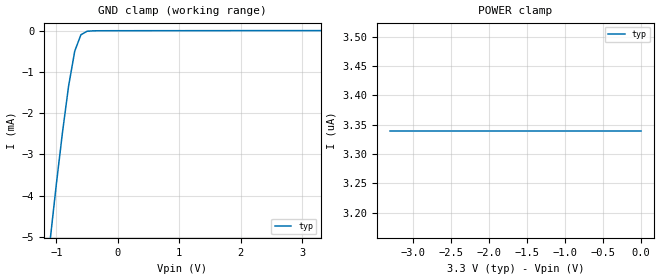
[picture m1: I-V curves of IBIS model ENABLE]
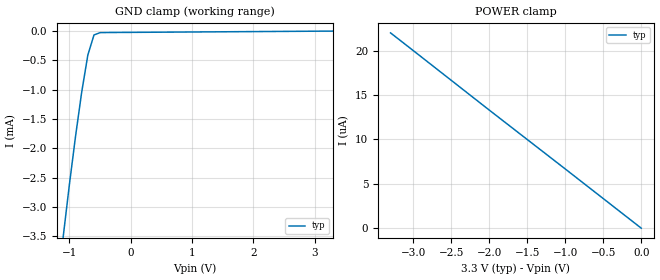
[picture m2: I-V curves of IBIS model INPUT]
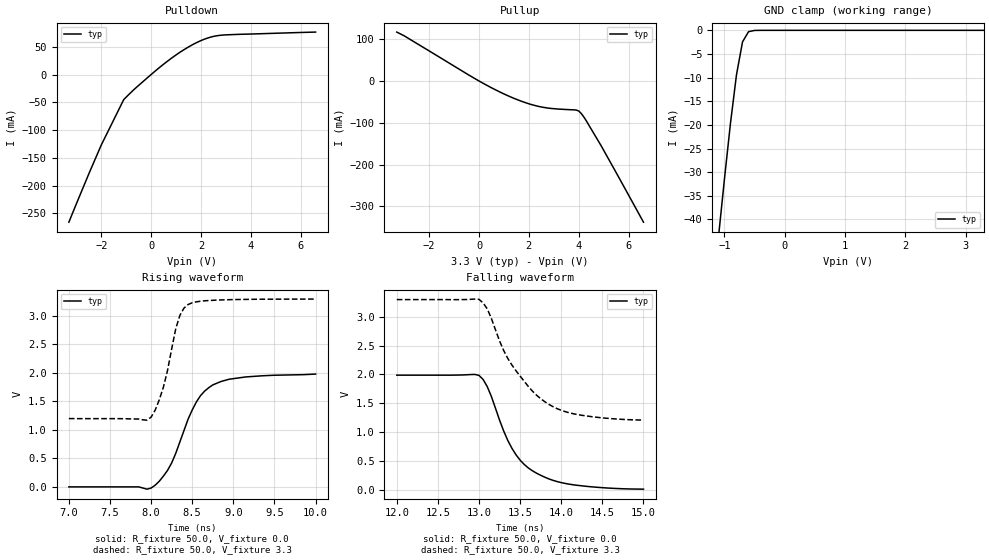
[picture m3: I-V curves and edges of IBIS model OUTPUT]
|   Texas Instruments Incorporated
|   Data Transmissions Products
|   IBIS Model for SN65LVDT386
|   64DGG TSSOP Package
[IBIS Ver]   2.1
[Comment char]   |_char
[File name]   lvdt386.ibs
[File Rev]   1.0
[Date]   28Jul99
[Source]   File originated at Texas Instruments Incorporated.
   Data Transmission Products Group.
[Notes]
[Disclaimer]
(C) Copyright Texas Instruments Incorporated 1999
   All rights reserved
  Texas Instruments Incorporated hereby grants the user of this IBIS
model a non-exclusive, nontransferable license to use this IBIS model
under the following terms.  Before using this IBIS model, the user
should read this license.  If the user does not accept these terms,
the IBIS model should be returned to Texas Instruments within 30 days.
  The user is granted this license only to use the IBIS model and
is not granted rights to sell, load, rent, lease or license the IBIS
model in whole or in part, or in modified form to anyone other than
user.  User may modify the IBIS model to suit its specific applications
but rights to derivative works and such modifications shall belong to
Texas Instruments.
  This IBIS model is provided on an "AS IS" basis and Texas Instruments
makes absolutely no warranty with respect to the information contained
herein.  TEXAS INSTRUMENTS DISCLAIMS AND CUSTOMER WAIVES ALL WARRANTIES,
EXPRESS OR IMPLIED, INCLUDING WARRANTIES OF MERCHANTABILITY OR FITNESS
FOR A PARTICULAR PURPOSE. The entire risk as to quality and performance
is with the Customer. ACCORDINGLY, IN NO EVENT SHALL THE COMPANY BE LIABLE
FOR ANY DAMAGES, WHETHER IN CONTRACT OR TORT,INCLUDING ANY LOST PROFITS
OR OTHER INCIDENTAL, CONSEQUENTIAL, EXEMPLARY, OR PUNITIVE DAMAGES ARISING
OUT OF THE USE OR APPLICATION OF THE IBIS model provided in this package.
Further, Texas Instruments reserves the right to discontinue or make changes
without notice to any product herein to improve reliability, function, or
design. Texas Instruments does not convey any license under patent rights
or any other intellectual property rights, including those of third parties.
Contact Texas Instruments at ATTN:DATA TRANSMISSIONS
Thomas Fisher 8505 Forest Lane, M/S 8710, Dallas, TX 75243-4136
[Copyright]   Copyright 1999, Texas Instruments, All Rights Reserved
[Component]   LVDT386DGG
[Manufacturer]  Texas Instruments Incorporated
[Package]
|   typ   min   max
R_pkg   0.068   0.046   0.094
L_pkg   3.798nH   2.565nH   5.991nH
C_pkg   0.564pF   0.297pF   1.022pF
[Pin]   signal_name   model_name   R_pin   L_pin   C_pin
1   A1A   INPUT   0.094   5.991n   0.940p
2   A1B   INPUT   0.090   5.514n   1.005p
3   A2A   INPUT   0.092   5.261n   0.912p
4   A2B   INPUT   0.092   4.891n   0.805p
5   A3A   INPUT   0.085   4.561n   0.702p
6   A3B   INPUT   0.084   4.247n   0.597p
7   A4A   INPUT   0.080   3.933n   0.534p
8   A4B   INPUT   0.077   3.622n   0.523p
9   B1A   INPUT   0.050   3.372n   0.483p
10   B1B   INPUT   0.048   3.139n   0.415p
11   B2A   INPUT   0.049   3.042n   0.397p
12   B2B   INPUT   0.051   2.941n   0.384p
13   B3A   INPUT   0.050   2.800n   0.355p
14   B3B   INPUT   0.052   2.711n   0.335p
15   B4A   INPUT   0.051   2.589n   0.314p
16   B4B   INPUT   0.055   2.604n   0.303p
17   C1A   INPUT   0.055   2.597n   0.302p
18   C1B   INPUT   0.052   2.605n   0.315p
19   C2A   INPUT   0.051   2.694n   0.334p
20   C2B   INPUT   0.050   2.772n   0.352p
21   C3A   INPUT   0.048   2.864n   0.372p
22   C3B   INPUT   0.049   2.982n   0.392p
23   C4A   INPUT   0.049   3.129n   0.413p
24   C4B   INPUT   0.046   3.263n   0.480p
25   D1A   INPUT   0.077   3.592n   0.542p
26   D1B   INPUT   0.081   3.923n   0.557p
27   D2A   INPUT   0.086   4.252n   0.614p
28   D2B   INPUT   0.085   4.525n   0.714p
29   D3A   INPUT   0.087   4.810n   0.813p
30   D3B   INPUT   0.089   5.135n   0.918p
31   D4A   INPUT   0.090   5.486n   1.019p
32   D4B   INPUT   0.090   5.912n   0.936p
33   GND   GND   0.087   5.926n   0.931p
34   VCC   POWER   0.087   5.496n   1.004p
35   VCC   POWER   0.087   5.124n   0.902p
36   GND   GND   0.088   4.867n   0.807p
37   END   ENABLE   0.086   4.514n   0.707p
38   D4Y   OUTPUT   0.085   4.206n   0.605p
39   D3Y   OUTPUT   0.089   3.929n   0.537p
40   D2Y   OUTPUT   0.079   3.584n   0.528p
41   D1Y   OUTPUT   0.048   3.299n   0.481p
42   ENC   ENABLE   0.048   3.101n   0.409p
43   C4Y   OUTPUT   0.048   2.969n   0.388p
44   C3Y   OUTPUT   0.048   2.855n   0.369p
45   C2Y   OUTPUT   0.049   2.766n   0.349p
46   C1Y   OUTPUT   0.051   2.696n   0.331p
47   GND   GND   0.052   2.638n   0.315p
48   VCC   POWER   0.053   2.565n   0.297p
49   VCC   POWER   0.052   2.574n   0.299p
50   GND   GND   0.051   2.617n   0.313p
51   B4Y   OUTPUT   0.050   2.666n   0.329p
52   B3Y   OUTPUT   0.050   2.769n   0.350p
53   B2Y   OUTPUT   0.049   2.909n   0.378p
54   B1Y   OUTPUT   0.048   2.993n   0.390p
55   ENB   ENABLE   0.049   3.176n   0.416p
56   A4Y   OUTPUT   0.048   3.295n   0.483p
57   A3Y   OUTPUT   0.079   3.569n   0.536p
58   A2Y   OUTPUT   0.082   3.908n   0.547p
59   A1Y   OUTPUT   0.086   4.238n   0.613p
60   ENA   ENABLE   0.086   4.509n   0.714p
61   GND   GND   0.089   4.863n   0.822p
62   VCC   POWER   0.090   5.197n   0.923p
63   VCC   POWER   0.092   5.558n   1.022p
64   GND   GND   0.090   5.947n   0.946p
[Diff_pin]   inv_pin   vdiff   tdelay_typ   tdelay_min   tdelay_max
| The 'xA' pin is Diff_pin and the 'xB' pin is the inv_pin
1   2   100   0 0 0
3   4   100   0 0 0
5   6   100   0 0 0
7   8   100   0 0 0
9   10   100   0 0 0
11   12   100   0 0 0
13   14   100   0 0 0
15   16   100   0 0 0
17   18   100   0 0 0
19   20   100   0 0 0
21   22   100   0 0 0
23   24   100   0 0 0
25   26   100   0 0 0
27   28   100   0 0 0
29   30   100   0 0 0
31   32   100   0 0 0
| Models and submodels in the file (3): ENABLE (Input), INPUT (Input), OUTPUT (3-state)
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|   Enable Model
[Model]   ENABLE
Model_type   Input
|Signals   ENA,ENB,ENC,END
Vinh = 2.0
Vinl = 0.8
|   typ   min   max
C_comp   1.0pF   NA   NA
|   typ   min   max
[Temperature Range]   25.0   NA   NA
[Voltage range]   3.3V   3.0V   3.6V
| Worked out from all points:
|   GND clamp passes 1 mA (typ) near -0.76 V on its own axis
[GND_clamp]
|   Voltage   I(typ)   I(min)   I(max)
-3.3V     -43.1mA    NA         NA
-1.1V     -5.08mA    NA         NA
-1V       -3.73mA    NA         NA
-900mV    -2.47mA    NA         NA
-800mV    -1.34mA    NA         NA
-700mV    -493uA     NA         NA
-600mV    -98.5uA    NA         NA
-500mV    -13.3uA    NA         NA
3.3V      3.34uA     NA         NA
[Power_clamp]
| Note that the[POWER_clamp]voltage table is referenced to Vcc
| and is calculated using Vtable=Vcc - Vmeasured.
|   Voltage   I(typ)   I(min)   I(max)
-3.3V     3.34uA     NA         NA
-2.7V     3.34uA     NA         NA
-2V       3.34uA     NA         NA
-800mV    3.34uA     NA         NA
0V        3.34uA     NA         NA
|   Receiver Input Model
[Model]   INPUT
Model_type   Input
|Signals   A1A,A1B,A2A,A2B,A3A,A3B,A4A,A4B,B1A,B1B,B2A,B2B,B3A,B3B,B4A,B4B
|   C1A,C1B,C2A,C2B,C3A,C3B,C4A,C4B,D1A,D1B,D2A,D2B,D3A,D3B,D4A,D4B
Vinh = 2.0
Vinl = 0.8
|   typ   min   max
C_comp   1.0pF   NA   NA
|   typ   min   max
[Temperature Range]   25.0   NA   NA
[Voltage range]   3.3V   3.0V   3.6V
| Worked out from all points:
|   GND clamp passes 1 mA (typ) near -0.79 V on its own axis
[GND_clamp]
|   Voltage   I(typ)   I(min)   I(max)
-3.3V     -32.7mA    NA         NA
-1.1V     -3.49mA    NA         NA
-1V       -2.61mA    NA         NA
-900mV    -1.79mA    NA         NA
-800mV    -1.04mA    NA         NA
-700mV    -409uA     NA         NA
-600mV    -66.6uA    NA         NA
-500mV    -26.4uA    NA         NA
3.3V      40.7pA     NA         NA
[Power_clamp]
| Note that the[POWER_clamp]voltage table is referenced to Vcc
| and is calculated using Vtable=Vcc - Vmeasured.
|   Voltage   I(typ)   I(min)   I(max)
-3.3V     22uA       NA         NA
-3V       20uA       NA         NA
-2V       13.3uA     NA         NA
-1V       6.67uA     NA         NA
0V        40.7pA     NA         NA
|   Receiver Output Model
[Model]   OUTPUT
Model_type   3-state
| Signals   A1Y,A2Y,B1Y,B2Y,C1Y,C2Y,D1Y,D2Y
Vmeas = 1.5V   |Reference voltage for timing measurements
Cref = 8pF   |Timing specification test load capacitance value
Vref = 0   |Timing specification test load voltage; GND
| variable   typ   min   max
C_comp   1.0pF   NA   NA
|   typ   min   max
[Temperature Range]   25.0   NA   NA
[Voltage range]   3.3V   3.0V   3.6V
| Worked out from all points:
|   slope of the pulldown table from 0 to 0.495 V, typ, clamps not added: 26.9 ohm
|   slope of the pullup table from 0 to 0.495 V, typ, clamps not added: 30.7 ohm
|   GND clamp passes 1 mA (typ) near -0.63 V on its own axis
|   rising waveform, R_fixture 50.0, V_fixture 0.0: 20-80 % time 352ps typ, NA min, NA max; typ from 0 V to 1.98 V
|   falling waveform, R_fixture 50.0, V_fixture 0.0: 20-80 % time 420ps typ, NA min, NA max; typ from 1.99 V to 0.006 V
|   rising waveform, R_fixture 50.0, V_fixture 3.3: 20-80 % time 202ps typ, NA min, NA max; typ from 1.2 V to 3.3 V
|   falling waveform, R_fixture 50.0, V_fixture 3.3: 20-80 % time 538ps typ, NA min, NA max; typ from 3.3 V to 1.21 V
[Pulldown]
|   Voltage   I(typ)   I(min)   I(max)
-3.3V     -266mA     NA         NA
-2.5V     -179mA     NA         NA
-2V       -127mA     NA         NA
-1.1V     -45.3mA    NA         NA
-600mV    -23.5mA    NA         NA
600mV     22.1mA     NA         NA
1.2V      41.4mA     NA         NA
1.7V      54.7mA     NA         NA
2.1V      63mA       NA         NA
2.5V      68.7mA     NA         NA
3V        71.5mA     NA         NA
6.6V      76.5mA     NA         NA
[Pullup]
|   Voltage   I(typ)   I(min)   I(max)
| Note that the[Pullup]voltage table is referenced to Vcc
| and is calculated using Vtable=Vcc - Vmeasured.
-3.3V     117mA      NA         NA
-3V       108mA      NA         NA
0V        1.74nA     NA         NA
1.3V      -39mA      NA         NA
1.9V      -52.6mA    NA         NA
2.4V      -61mA      NA         NA
3.9V      -69.6mA    NA         NA
4V        -71.8mA    NA         NA
4.1V      -77.6mA    NA         NA
4.3V      -94.9mA    NA         NA
4.9V      -155mA     NA         NA
6.6V      -338mA     NA         NA
[GND_clamp]
|   Voltage   I(typ)   I(min)   I(max)
| Outputs in High Impedance (off)
-3.3V     -346mA     NA         NA
-1.1V     -43.9mA    NA         NA
-1V       -31.5mA    NA         NA
-900mV    -19.7mA    NA         NA
-800mV    -9.41mA    NA         NA
-700mV    -2.45mA    NA         NA
-600mV    -285uA     NA         NA
-400mV    -1.52uA    NA         NA
3.3V      489pA      NA         NA
[POWER_clamp]
|   Voltage   I(typ)   I(min)   I(max)
| Note that the [POWER_clamp] voltage table is referenced to Vcc
| and is calculated using Vtable = Vcc - Vmeasured.
| Outputs in Tri-state.
-3.3V     0A         NA         NA
0V        0A         NA         NA
[Ramp]
|   typ   min   max
dV/dt_r   1.20V/353ps   NA   NA
dV/dt_f   1.26V/540ps   NA   NA
R_load = 50
[Rising Waveform]
R_fixture = 50.0
V_fixture = 0.0
C_fixture = 0p
L_fixture = 0n
|   V(typ)   V(min)   V(max)
7ns       0V         NA         NA
8ns       -20mV      NA         NA
8.2ns     290mV      NA         NA
8.3ns     590mV      NA         NA
8.5ns     1.35V      NA         NA
8.6ns     1.6V       NA         NA
8.7ns     1.74V      NA         NA
8.85ns    1.85V      NA         NA
9.15ns    1.93V      NA         NA
10ns      1.98V      NA         NA
[Falling Waveform]
R_fixture = 50.0
V_fixture = 0.0
C_fixture = 0p
L_fixture = 0n
|   V(typ)   V(min)   V(max)
12ns      1.986V     NA         NA
13ns      1.982V     NA         NA
13.1ns    1.787V     NA         NA
13.3ns    1.016V     NA         NA
13.4ns    716mV      NA         NA
13.5ns    510mV      NA         NA
13.6ns    374mV      NA         NA
13.85ns   184mV      NA         NA
14.05ns   105mV      NA         NA
15ns      6mV        NA         NA
[Rising Waveform]
R_fixture = 50.0
V_fixture = 3.3
C_fixture = 0p
L_fixture = 0n
|   V(typ)   V(min)   V(max)
7ns       1.199V     NA         NA
7.95ns    1.171V     NA         NA
8ns       1.224V     NA         NA
8.05ns    1.349V     NA         NA
8.15ns    1.753V     NA         NA
8.3ns     2.778V     NA         NA
8.35ns    3.011V     NA         NA
8.45ns    3.201V     NA         NA
8.8ns     3.279V     NA         NA
10ns      3.297V     NA         NA
[Falling Waveform]
R_fixture = 50.0
V_fixture = 3.3
C_fixture = 0p
L_fixture = 0n
|   V(typ)   V(min)   V(max)
12ns      3.299V     NA         NA
13ns      3.303V     NA         NA
13.1ns    3.138V     NA         NA
13.25ns   2.58V      NA         NA
13.35ns   2.276V     NA         NA
13.6ns    1.789V     NA         NA
13.75ns   1.577V     NA         NA
13.95ns   1.404V     NA         NA
14.15ns   1.315V     NA         NA
15ns      1.206V     NA         NA
